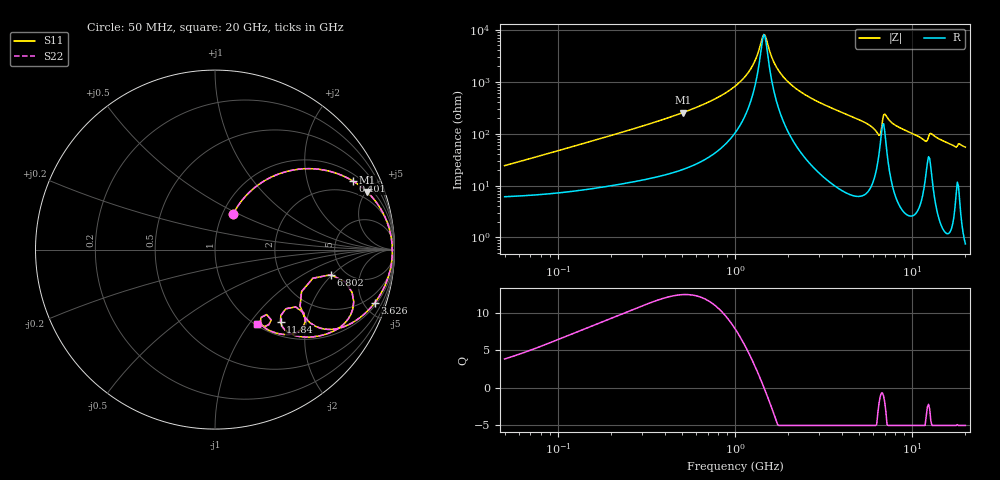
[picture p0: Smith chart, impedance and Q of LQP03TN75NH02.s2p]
!Murata Part Number: LQP03TN75NH02
!These Parameters are Measured in Series Mode Connection
!  o--[Z]--o
!Port1  Port2
!  o-------o
!Freq. Start=50[MHz] Stop=20[GHz], 401[Steps]
# Hz S RI R 50
!Freq.(Hz) S11(Real) S11(Imag) S21(Real) S21(Imag) S12(Real) S12(Imag) S22(Real) S22(Imag)
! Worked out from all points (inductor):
!   401 points, 50 MHz to 20 GHz, reference 50 ohm
!   read as one part in series: L = 74 nH near 51.52 MHz
!   highest Q = 12.4 at 509.6 MHz (marker M1), where L = 79.4 nH
!   self-resonance near 1.454 GHz
!   S11 on the Smith chart (normalised r, x): 50 MHz: 1.12, +0.47; 401 MHz: 1.32, +3.82; 3.626 GHz: 1.20, -5.93; 6.802 GHz: 3.87, -1.92; 11.84 GHz: 1.24, -1.43; 20 GHz: 1.02, -1.10
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5e7  0.1012 0.1984  0.8988 -0.1984  0.8988 -0.1984  0.1012 0.1984
1.364002e8  0.3086 0.4015  0.6914 -0.4015  0.6914 -0.4015  0.3086 0.4015
3.721004e8  0.7393 0.3985  0.2607 -0.3985  0.2607 -0.3985  0.7393 0.3985
4.010383e8  0.768 0.3824  0.232 -0.3824  0.232 -0.3824  0.768 0.3824
5.096456e8  0.8479 0.3211  0.1521 -0.3211  0.1521 -0.3211  0.8479 0.3211
1e9  0.9709 0.1162  0.0291 -0.1162  0.0291 -0.1162  0.9709 0.1162
1.23331e9  0.9841 0.0517  0.0159 -0.0517  0.0159 -0.0517  0.9841 0.0517
1.454215e9  0.9879 0.00112  0.0121 -0.00112  0.0121 -0.00112  0.9879 0.00112
1.498439e9  0.988 -0.00809  0.012 0.00809  0.012 0.00809  0.988 -0.00809
1.664083e9  0.9869 -0.0405  0.0131 0.0405  0.0131 0.0405  0.9869 -0.0405
1.848039e9  0.9834 -0.0732  0.0166 0.0732  0.0166 0.0732  0.9834 -0.0732
2.728004e9  0.9475 -0.1993  0.0525 0.1993  0.0525 0.1993  0.9475 -0.1993
3.626126e9  0.89 -0.2964  0.11 0.2964  0.11 0.2964  0.89 -0.2964
5.944466e9  0.6316 -0.4447  0.3684 0.4447  0.3684 0.4447  0.6316 -0.4447
6.503449e9  0.4741 -0.3142  0.5259 0.3142  0.5259 0.3142  0.4741 -0.3142
6.802353e9  0.645 -0.1402  0.355 0.1402  0.355 0.1402  0.645 -0.1402
7.114996e9  0.773 -0.2908  0.227 0.2908  0.227 0.2908  0.773 -0.2908
7.442007e9  0.7424 -0.386  0.2576 0.386  0.2576 0.386  0.7424 -0.386
9.745021e9  0.5253 -0.4872  0.4747 0.4872  0.4747 0.4872  0.5253 -0.4872
1.183995e10  0.3651 -0.4036  0.6349 0.4036  0.6349 0.4036  0.3651 -0.4036
1.295331e10  0.4898 -0.433  0.5102 0.433  0.5102 0.433  0.4898 -0.433
2e10  0.2344 -0.4168  0.7656 0.4168  0.7656 0.4168  0.2344 -0.4168
